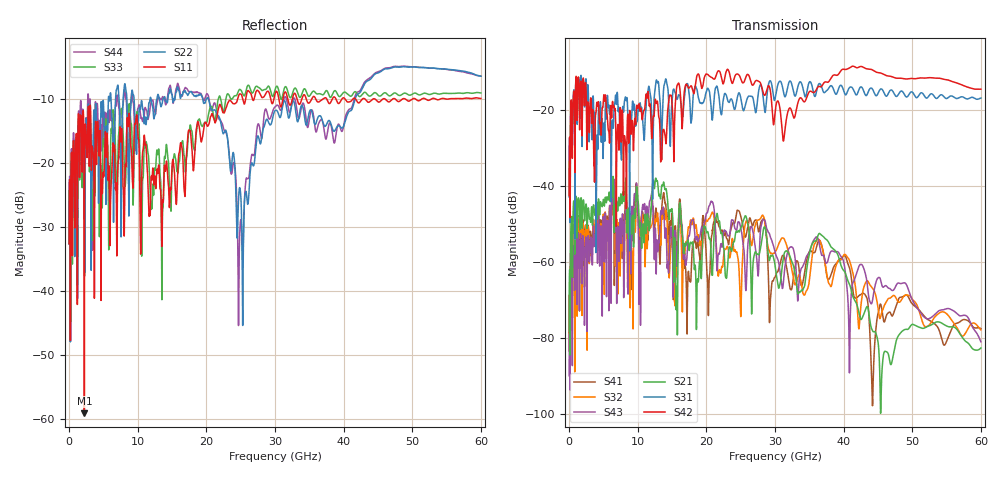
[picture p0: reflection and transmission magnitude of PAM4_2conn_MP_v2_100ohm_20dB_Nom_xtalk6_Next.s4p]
! Info: Touchstone file created by Circ.  Input file=FAB50GbE_2conn_Midplane_Examax_Topo2_v2_100ohm_20dB_Nom.circ
# Hz S RI R 50
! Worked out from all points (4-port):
!   6000 points, 10 MHz to 60 GHz, reference 50 ohm
!   strongest paths, dB at 10 MHz, 15.01 GHz, 30.01 GHz, 45.01 GHz, 60 GHz:
!     S42: -42.6, -18.4, -20.8, -10.2, -14.6
!     S31: -42.9, -17.5, -17.1, -15.7, -16.9
!     S21: -78.3, -46.3, -60.9, -81.1, -82.7
!     S43: -90.0, -53.6, -57.4, -64.2, -81.1
!     S32: -78.7, -53.8, -57.5, -72.1, -78.0
!     S41: -83.4, -47.4, -64.1, -73.7, -77.6
!   lowest |S11| = -59.2 dB at 2.23 GHz (marker M1), VSWR 1.00, Z = 49.9 - j0.0225 ohm
!   |S11| at or under -10 dB: start of sweep to 24.55 GHz; 40.24 GHz to 41.32 GHz (1.083 GHz wide, 2.66 % of centre); 43.16 GHz to 44.21 GHz (1.054 GHz wide, 2.41 % of centre)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
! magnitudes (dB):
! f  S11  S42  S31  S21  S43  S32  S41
! 10 MHz  -32.6  -42.6  -42.9  -78.3  -90.0  -78.7  -83.4
! 2.23 GHz  -59.2  -18.7  -18.1  -48.3  -67.9  -64.2  -61.3
! 20.13 GHz  -14.2  -10.7  -14.5  -52.1  -47.1  -49.3  -63.6
! 24.87 GHz  -9.2  -11.1  -15.8  -51.9  -50.0  -66.6  -47.1
! 28.16 GHz  -9.7  -14.6  -14.9  -53.4  -49.3  -47.8  -49.0
! 29.36 GHz  -9.8  -15.4  -12.4  -58.4  -53.6  -57.9  -69.4
! 60 GHz  -9.9  -14.6  -16.9  -82.7  -81.1  -78.0  -77.6
